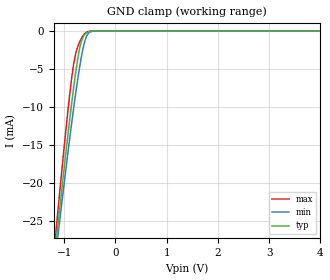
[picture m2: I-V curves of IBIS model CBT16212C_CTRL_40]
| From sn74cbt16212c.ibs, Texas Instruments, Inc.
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[Model]   CBT16212C_CTRL_40
Model_type  Input
Vinl=0.8
Vinh=2.0
| variable   typ   min   max
C_comp   2.55pF   1.92pF   3.26pF
[Temperature Range]   40   100   -40
| Ambient temperature   25   85   -40
[Voltage range]   4   4   4
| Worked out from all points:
|   GND clamp passes 1 mA (typ) near -0.64 V on its own axis
[GND Clamp]
| CBT16212C_CTRL_40
|   Voltage   I(typ)   I(min)   I(max)
-4V       -228.8mA   -212.9mA   -247.5mA
-1.17V    -28.74mA   -29.84mA   -27.17mA
-1.135V   -26.51mA   -27.8mA    -24.68mA
-1.105V   -24.62mA   -26.07mA   -22.57mA
-920mV    -13.37mA   -15.72mA   -10.16mA
-815mV    -7.538mA   -10.24mA   -4.411mA
-765mV    -5.061mA   -7.792mA   -2.746mA
-680mV    -1.807mA   -4.063mA   -1.206mA
-615mV    -615.7uA   -1.842mA   -472.5uA
-555mV    -205.1uA   -602.7uA   -131.7uA
-410mV    -6.4uA     -14.18uA   -1.367uA
4V        94.32pA    243.3pA    55.56pA
